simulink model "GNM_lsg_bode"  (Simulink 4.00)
settings: Solver=ode45  StartTime=0.0  StopTime=0.2  FixedStep=0.005  RelTol=1e-3
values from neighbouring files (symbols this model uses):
  CE = (2*NA/pi)*2*pi    (= 240)    [GNM_lsg_ini.m]
  CM = 2*NA/pi    (= 38.1971863421)    [GNM_lsg_ini.m]
  Fpwm = 5000    [GNM_lsg_ini.m]
  J = 0.012    [GNM_lsg_ini.m]
  LA = 0.004    [GNM_lsg_ini.m]
  psi = 0.04    [GNM_lsg_ini.m]
  RA = 0.25    [GNM_lsg_ini.m]
  Umax = 200    [GNM_lsg_ini.m]
libraries: simulink3 x1

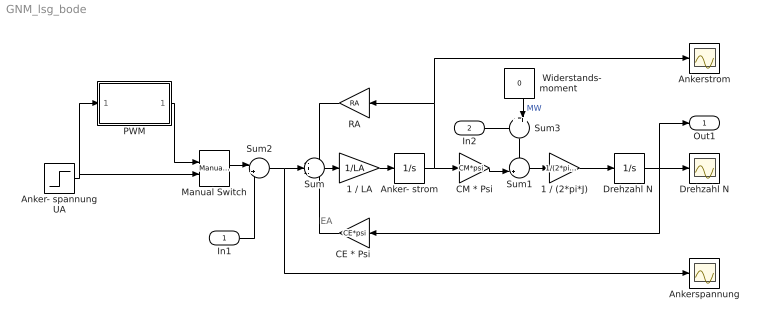
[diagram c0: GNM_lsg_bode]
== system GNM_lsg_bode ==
  note: EA
  In1 : Inport  Port=1
  In2 : Inport  Port=2
  " Widerstands-  moment" : Constant  Orientation=down  Value=0
  1 / (2*pi*J) : Gain  Gain=1/(2*pi*J)  Multiplication=Element-wise(K.*u)  SaturateOnIntegerOverflow=on
  1 / LA : Gain  Gain=1/LA  Multiplication=Element-wise(K.*u)  SaturateOnIntegerOverflow=on
  Anker- spannung UA : Step  Time=0.05  Before=0  After=50  SampleTime=0
  Anker- strom : Integrator  ExternalReset=none  InitialConditionSource=internal  InitialCondition=0  LimitOutput=off  UpperSaturationLimit=inf  LowerSaturationLimit=-inf  ShowSaturationPort=off  ShowStatePort=off  AbsoluteTolerance=auto
  Ankerspannung : Scope
  Ankerstrom : Scope
  "CE * Psi " : Gain  Orientation=left  Gain=CE*psi  Multiplication=Element-wise(K.*u)  SaturateOnIntegerOverflow=on
  CM * Psi : Gain  Gain=CM*psi  Multiplication=Element-wise(K.*u)  SaturateOnIntegerOverflow=on
  Drehzahl N : Scope
  "Drehzahl N " : Integrator  ExternalReset=none  InitialConditionSource=internal  InitialCondition=0  LimitOutput=off  UpperSaturationLimit=inf  LowerSaturationLimit=-inf  ShowSaturationPort=off  ShowStatePort=off  AbsoluteTolerance=auto
  Manual Switch : simulink3/Nonlinear/Manual Switch  sw=0  action=0
  PWM : Subsystem
  RA : Gain  Orientation=left  Gain=RA  Multiplication=Element-wise(K.*u)  SaturateOnIntegerOverflow=on
  Sum : Sum  Inputs=-+-  SaturateOnIntegerOverflow=on
  Sum1 : Sum  Inputs=-+|  SaturateOnIntegerOverflow=on
  Sum2 : Sum  Inputs=|++  SaturateOnIntegerOverflow=on
  Sum3 : Sum  Orientation=down  Inputs=++|  SaturateOnIntegerOverflow=on
  Out1 : Outport  Port=1
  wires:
  PWM/1(UAist) -> Manual Switch/1
  Anker- spannung UA/1 -> PWM/1(UAsoll), Manual Switch/2
  In1/1 -> Sum2/2
  Manual Switch/1 -> Sum2/1
  RA/1 -> Sum/1
  Anker- strom/1 -> CM * Psi/1, RA/1, Ankerstrom/1
  Sum/1 -> 1 / LA/1
  1 / LA/1 -> Anker- strom/1
  CM * Psi/1 -> Sum1/2
  Sum1/1 -> 1 / (2*pi*J)/1
  1 / (2*pi*J)/1 -> "Drehzahl N "/1
  "CE * Psi "/1 -> Sum/3
  "Drehzahl N "/1 -> "CE * Psi "/1, Drehzahl N/1, Out1/1
  Sum2/1 -> Sum/2, Ankerspannung/1
  Sum3/1 -> Sum1/1
  In2/1 -> Sum3/1
  " Widerstands-  moment"/1 -> Sum3/2  "MW"

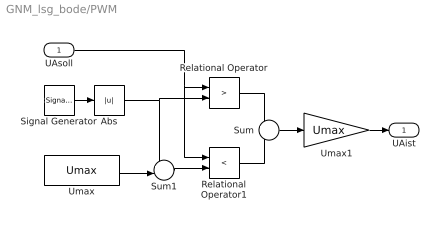
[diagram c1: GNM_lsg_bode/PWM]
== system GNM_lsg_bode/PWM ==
  UAsoll : Inport  Port=1
  Abs : Abs  SaturateOnIntegerOverflow=on
  Relational Operator : RelationalOperator  Operator=>
  Relational Operator1 : RelationalOperator  Operator=<
  Signal Generator : SignalGenerator  WaveForm=sawtooth  Amplitude=Umax  Frequency=Fpwm  Units=Hertz
  Sum : Sum  Inputs=+-  SaturateOnIntegerOverflow=on
  Sum1 : Sum  Inputs=+-|  SaturateOnIntegerOverflow=on
  Umax : Constant  Value=Umax
  Umax1 : Gain  Gain=Umax  Multiplication=Element-wise(K.*u)  SaturateOnIntegerOverflow=on
  UAist : Outport  Port=1  InitialOutput=0
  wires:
  Sum/1 -> Umax1/1
  Umax1/1 -> UAist/1
  Relational Operator1/1 -> Sum/2
  Relational Operator/1 -> Sum/1
  Umax/1 -> Sum1/2
  Abs/1 -> Sum1/1, Relational Operator/2
  UAsoll/1 -> Relational Operator/1, Relational Operator1/1
  Sum1/1 -> Relational Operator1/2
  Signal Generator/1 -> Abs/1
